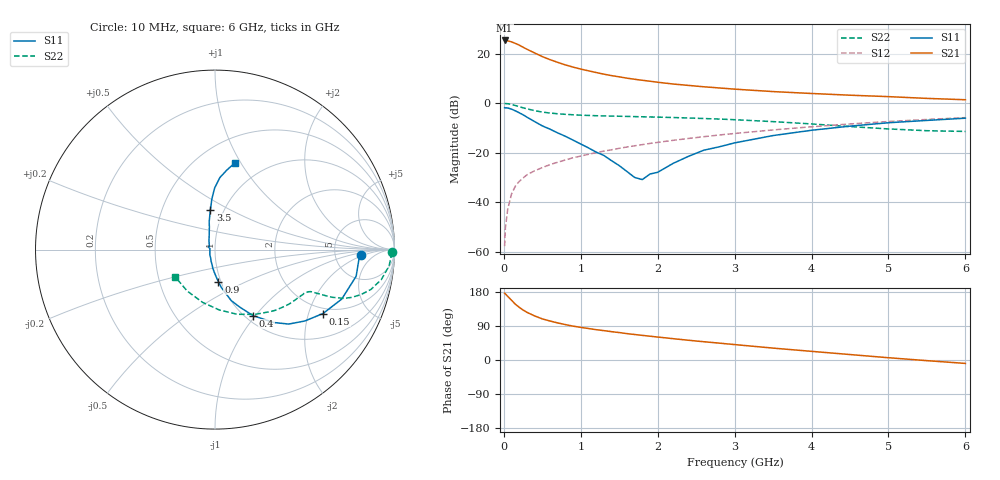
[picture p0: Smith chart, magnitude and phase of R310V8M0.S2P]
! SIEMENS Small Signal Semiconductors
! BFR181
! Si NPN RF Bipolar Junction Transistor in SOT23
! VCE = 10 V  IC = 8 mA
! Common Emitter S-Parameters:  May  1996
# GHz  S  MA  R  50
!  f  S11  S21  S12  S22
! GHz  MAG  ANG  MAG  ANG  MAG  ANG  MAG  ANG
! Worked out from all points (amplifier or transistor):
!   36 points, 10 MHz to 6 GHz, reference 50 ohm
!   highest |S21| = 25.3 dB at 10 MHz (marker M1)
!   |S21| within 3 dB of that: start of sweep to 266.8 MHz
!   unconditionally stable (mu >= 1): 993.1 MHz to 2.969 GHz
!   at 250 MHz: K = 0.52, MSG = 26.4 dB, |S12| = -30.2 dB
!   at 1.4 GHz: K = 1.04, MAG = 13.7 dB, |S12| = -18.8 dB
!   at 6 GHz: K = 0.87, MSG = 3.6 dB, |S12| = -5.8 dB
!   S11 on the Smith chart (normalised r, x): 10 MHz: 9.32, -1.62; 150 MHz: 1.79, -2.50; 400 MHz: 1.08, -0.97; 900 MHz: 0.97, -0.36; 3.5 GHz: 0.86, +0.40; 6 GHz: 0.74, +0.95
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0.01  0.8115 -2.1  18.43 176.3  0.0013 80.0  0.9835 -0.9
0.02  0.8034 -4.1  18.09 174.4  0.003 85.9  0.9824 -2.2
0.05  0.8003 -10.7  18.11 168.1  0.0072 82.1  0.974 -5.4
0.1  0.7581 -21.3  17.26 157.7  0.0147 78.4  0.9417 -10.2
0.15  0.6994 -30.6  16.05 147.2  0.0212 74.4  0.8971 -14.3
0.2  0.6391 -38.5  14.84 138.9  0.0264 72.6  0.8501 -17.2
0.25  0.5836 -45.3  13.46 131.9  0.0308 69.3  0.8057 -19.3
0.3  0.5221 -51.1  12.25 125.8  0.0358 68.2  0.7689 -20.7
0.4  0.4251 -60.0  10.31 116.4  0.0432 66.7  0.7066 -22.1
0.5  0.348 -66.8  8.712 108.5  0.0501 67.4  0.6609 -22.7
0.6  0.2985 -72.3  7.556 102.9  0.0574 67.3  0.6321 -23.0
0.7  0.2511 -76.2  6.662 97.8  0.0643 67.5  0.6108 -23.3
0.9  0.1796 -83.9  5.342 89.4  0.0792 67.5  0.5826 -23.7
1.1  0.1251 -92.0  4.496 83.1  0.0929 67.8  0.5651 -24.8
1.4  0.0691 -108.3  3.597 74.8  0.1146 67.2  0.5493 -27.2
1.8  0.0287 169.6  2.897 65.0  0.1456 65.7  0.5312 -31.1
2.2  0.0609 123.5  2.436 56.3  0.1777 63.3  0.513 -36.1
2.6  0.1124 106.4  2.141 48.2  0.2107 60.6  0.4896 -41.7
3.5  0.222 96.7  1.712 31.4  0.2882 53.1  0.4241 -58.3
4.5  0.3439 90.3  1.448 14.4  0.3804 42.8  0.3367 -86.1
5.5  0.4484 81.5  1.248 -1.7  0.4691 30.7  0.278 -123.9
6  0.4974 76.9  1.172 -9.0  0.5107 24.1  0.2688 -145.5
